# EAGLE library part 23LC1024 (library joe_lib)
23LC1024 QSPI 1Mbit SRAM 1Mbit Serial SRAM
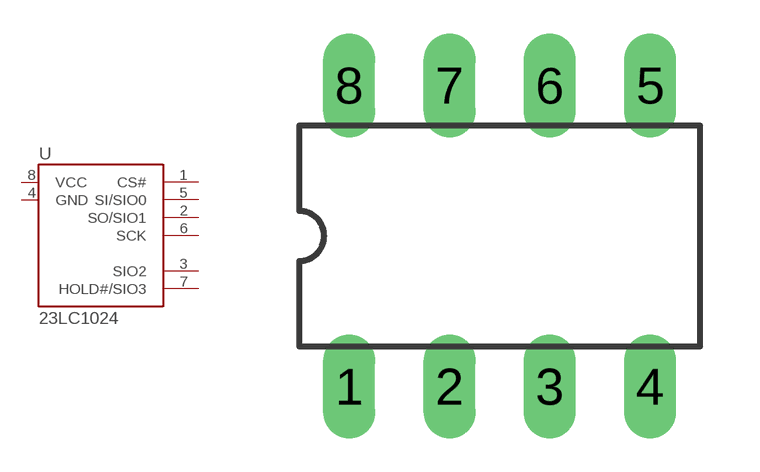
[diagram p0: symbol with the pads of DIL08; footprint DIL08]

Designator prefix U

## 23LC1024DIP  [DIL08]
1  CS#  in
2  SO/SIO1
3  SIO2
4  GND  pwr
5  SI/SIO0
6  SCK  in
7  HOLD#/SIO3
8  VCC  pwr

## Footprint DIL08 (pad centres in mm)
Dual In Line
drill 0.813 long: 1 -3.81,-3.81; 2 -1.27,-3.81; 3 1.27,-3.81; 4 3.81,-3.81; 5 3.81,3.81; 6 1.27,3.81; 7 -1.27,3.81; 8 -3.81,3.81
